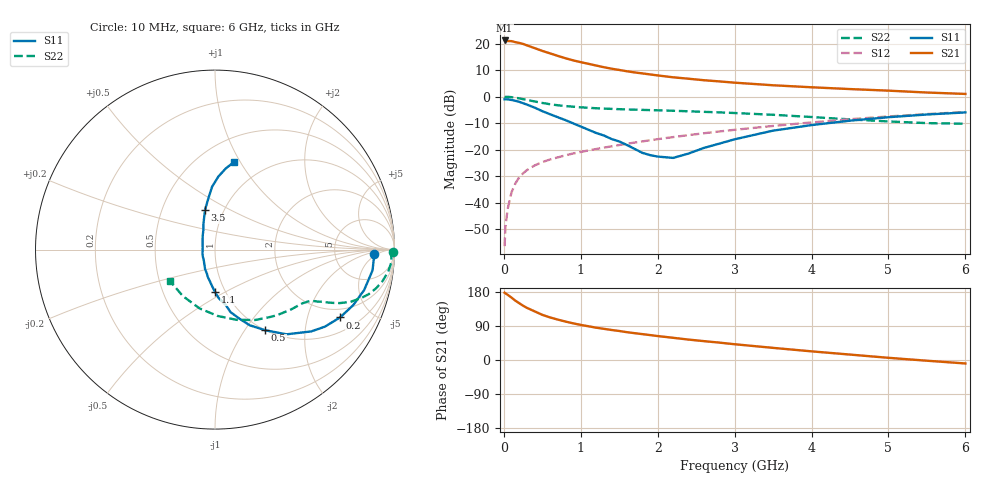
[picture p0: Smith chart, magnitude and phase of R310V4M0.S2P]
! SIEMENS Small Signal Semiconductors
! BFR181
! Si NPN RF Bipolar Junction Transistor in SOT23
! VCE = 10 V  IC = 4 mA
! Common Emitter S-Parameters:  May  1996
# GHz  S  MA  R  50
!  f  S11  S21  S12  S22
! GHz  MAG  ANG  MAG  ANG  MAG  ANG  MAG  ANG
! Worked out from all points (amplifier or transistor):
!   36 points, 10 MHz to 6 GHz, reference 50 ohm
!   highest |S21| = 21.2 dB at 10 MHz (marker M1)
!   |S21| within 3 dB of that: start of sweep to 410.8 MHz
!   unconditionally stable (mu >= 1): 1.301 GHz to 3.216 GHz
!   at 250 MHz: K = 0.36, MSG = 24.4 dB, |S12| = -29.0 dB
!   at 1.4 GHz: K = 1.02, MAG = 13.8 dB, |S12| = -18.8 dB
!   at 6 GHz: K = 0.86, MSG = 3.4 dB, |S12| = -5.8 dB
!   S11 on the Smith chart (normalised r, x): 10 MHz: 16, -4; 200 MHz: 1.58, -3.22; 500 MHz: 1.00, -1.25; 1.1 GHz: 0.90, -0.45; 3.5 GHz: 0.82, +0.38; 6 GHz: 0.72, +0.95
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0.01  0.8867 -1.6  11.42 177.6  0.0015 89.0  0.9938 -0.7
0.02  0.8867 -3.0  11.21 176.1  0.0034 83.0  0.9813 -1.5
0.05  0.8854 -7.5  11.15 172.0  0.0076 84.6  0.9867 -3.8
0.1  0.8609 -15.2  11.09 164.6  0.0156 83.1  0.9727 -7.3
0.15  0.8299 -21.9  10.61 156.6  0.0229 76.9  0.9494 -10.7
0.2  0.7925 -28.5  10.27 149.9  0.0299 73.7  0.9232 -13.5
0.25  0.7481 -35.0  9.826 143.3  0.0355 70.7  0.8912 -16.2
0.3  0.7035 -40.4  9.227 137.6  0.0409 69.4  0.8601 -18.2
0.4  0.6178 -49.8  8.194 128.4  0.05 65.7  0.8073 -21.2
0.5  0.5293 -58.1  7.259 119.2  0.0578 63.6  0.7565 -23.2
0.6  0.4635 -65.4  6.528 112.4  0.0648 62.6  0.7155 -24.5
0.7  0.4073 -70.6  5.85 106.7  0.0709 62.3  0.6839 -25.4
0.8  0.359 -76.0  5.279 101.5  0.0776 61.3  0.6602 -26.1
0.9  0.3117 -79.3  4.814 96.8  0.0841 61.0  0.6425 -26.8
1.1  0.2359 -89.9  4.14 89.0  0.0962 61.5  0.6122 -28.0
1.3  0.1841 -98.1  3.573 82.3  0.1088 61.7  0.5914 -29.3
1.6  0.1217 -116.9  2.995 73.4  0.1284 61.8  0.571 -31.7
2.2  0.0694 171.4  2.304 58.6  0.1715 60.5  0.5384 -38.4
3.5  0.2271 104.2  1.63 32.0  0.2784 52.9  0.4522 -60.1
4.5  0.35 92.7  1.382 14.3  0.3727 43.4  0.37 -87.7
5.5  0.4576 82.3  1.189 -1.9  0.4664 31.6  0.3148 -124.7
6  0.5012 77.5  1.119 -9.2  0.5103 24.8  0.3064 -145.6
